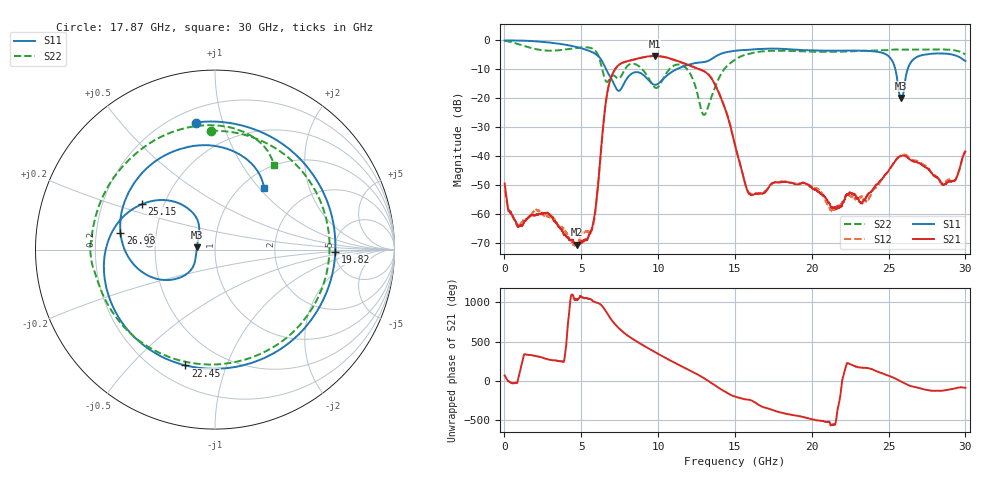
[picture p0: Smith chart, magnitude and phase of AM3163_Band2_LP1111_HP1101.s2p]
!Agilent Technologies,E8364B,MY43040894,A.07.50.67
!Agilent E8364B: A.07.50.67
!Date: Thursday, August 20, 2020 12:08:48
!Correction: S11(Full 2 Port(1,2))
!S21(Full 2 Port(1,2))
!S12(Full 2 Port(1,2))
!S22(Full 2 Port(1,2))
!S2P File: Measurements: S11, S21, S12, S22:
# Hz S  dB  R 50
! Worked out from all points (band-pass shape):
!   3201 points, 10 MHz to 30 GHz, reference 50 ohm
!   highest |S21| = -5.41 dB at 9.766 GHz (marker M1); lowest = -70.5 dB at 4.743 GHz (marker M2)
!   |S21| within 3 dB of the highest: 7.459 GHz to 11.93 GHz (4.47 GHz wide, 46.1 % of centre)
!   lowest |S11| = -19.9 dB at 25.83 GHz (marker M3), VSWR 1.23, Z = 40.9 + j0.994 ohm
!   |S11| at or under -10 dB: 6.613 GHz to 11.19 GHz (4.582 GHz wide, 51.5 % of centre); 25.44 GHz to 26.24 GHz (796.3 MHz wide, 3.08 % of centre)
!   |S22| runs from -25.7 to -0.2 dB; largest |S21 - S12| = 0.01
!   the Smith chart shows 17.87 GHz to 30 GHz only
!   S11 on the Smith chart (normalised r, x): 17.87 GHz: 0.28, +0.82; 19.82 GHz: 5.06, -0.20; 22.45 GHz: 0.31, -0.73; 25.15 GHz: 0.38, +0.25; 26.98 GHz: 0.30, +0.08; 30 GHz: 1.25, +1.07
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1e7  -0.05 -2.7  -49.43 70.4  -51.72 31.7  -0.16 -6.8
1.95935e9  -0.32 -72.9  -60.35 -40.7  -58.66 -42.3  -2.94 -171.3
3.3089e9  -1.00 -124.7  -62.43 -98.4  -62.24 -94.9  -3.53 88.8
4.742797e9  -2.37 173.6  -70.54 -49.5  -69.91 -34.7  -2.57 -7.7
5.014581e9  -2.75 159.9  -69.70 -14.4  -66.80 21.3  -2.43 -26.0
5.801819e9  -4.33 111.4  -62.28 -71.2  -62.98 -78.6  -3.11 -86.2
6.982675e9  -13.47 16.7  -12.18 52.3  -12.24 52.3  -12.40 -98.0
8.388456e9  -11.20 -83.8  -6.66 168.2  -6.71 168.5  -8.08 -128.2
9.766122e9  -15.33 173.6  -5.41 9.9  -5.41 10.0  -16.17 -161.1
1.000979e10  -14.96 168.6  -5.46 -16.6  -5.46 -16.7  -16.10 -145.8
1.144369e10  -9.41 61.7  -7.45 -164.5  -7.59 -163.5  -8.41 157.7
1.299942e10  -7.49 -43.2  -10.70 34.4  -10.67 35.8  -25.74 -96.1
1.5005e10  -3.60 -130.7  -36.22 162.2  -36.10 161.7  -6.69 -112.2
1.787279e10  -2.90 98.5  -49.01 -34.1  -48.90 -33.0  -3.58 92.0
1.982214e10  -3.47 -1.0  -50.12 -114.9  -49.99 -114.9  -3.91 -1.4
2.000958e10  -3.50 -9.7  -50.92 -123.6  -50.58 -122.6  -3.93 -9.5
2.244627e10  -3.53 -104.3  -52.60 -141.4  -53.65 -151.7  -3.83 -97.8
2.500479e10  -5.49 157.8  -44.89 67.7  -45.00 68.5  -3.36 -167.6
2.515474e10  -6.38 148.2  -43.73 55.9  -43.81 58.3  -3.27 -171.4
2.582952e10  -19.90 173.2  -39.95 -9.2  -39.54 -9.1  -3.21 170.0
2.698226e10  -5.43 169.8  -42.34 -88.5  -41.91 -88.2  -3.19 140.4
3e10  -7.14 51.4  -38.43 -86.3  -38.11 -85.8  -4.80 55.2
